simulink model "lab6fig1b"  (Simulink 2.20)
settings: Solver=ode45  StartTime=0.0  StopTime=10.0  RelTol=1e-3  AbsTol=1e-6

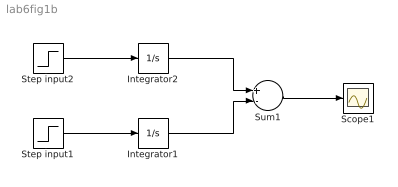
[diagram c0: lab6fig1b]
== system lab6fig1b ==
  Integrator1 : Integrator  ExternalReset=none  InitialConditionSource=internal  InitialCondition=0  LimitOutput=off  UpperSaturationLimit=inf  LowerSaturationLimit=-inf  ShowSaturationPort=off  ShowStatePort=off  AbsoluteTolerance=auto
  Integrator2 : Integrator  ExternalReset=none  InitialConditionSource=internal  InitialCondition=0  LimitOutput=off  UpperSaturationLimit=inf  LowerSaturationLimit=-inf  ShowSaturationPort=off  ShowStatePort=off  AbsoluteTolerance=auto
  Scope1 : Scope
  Step input1 : Step  Time=1  Before=0  After=1
  Step input2 : Step  Time=0  Before=0  After=1
  Sum1 : Sum  Inputs=+-
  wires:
  Integrator2/1 -> Sum1/1
  Integrator1/1 -> Sum1/2
  Step input2/1 -> Integrator2/1
  Step input1/1 -> Integrator1/1
  Sum1/1 -> Scope1/1
